TYPE ConfigMfcVer :
STRUCT
	BasePressure:SVLREAL;
	PumpingTime:SVINT;
	GasFlowTime:SVINT;
	HoldTime:SVINT;
	TargetPressure:SVLREAL;
	MaxDeviation:SVLREAL;
	PressureStableTolerance:SVLREAL;
	FlowStableTolerance:SVLREAL;
END_STRUCT
END_TYPE
